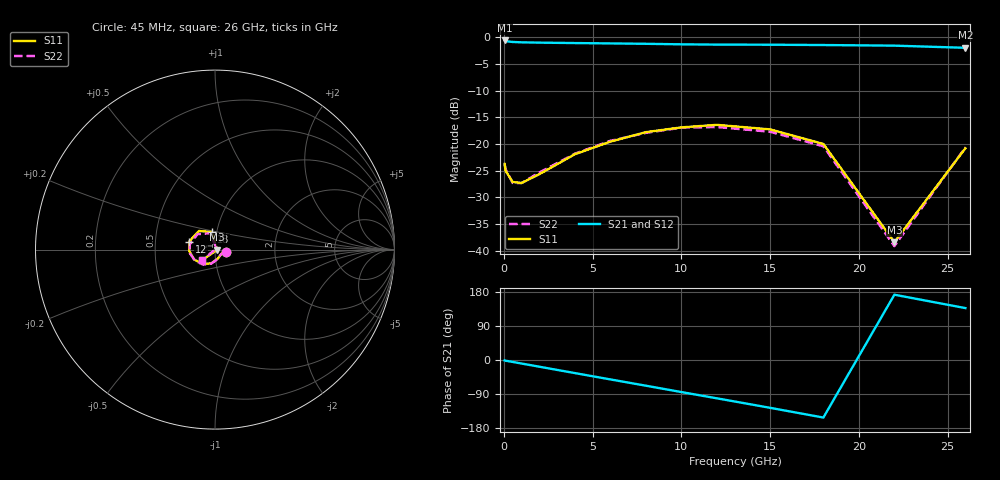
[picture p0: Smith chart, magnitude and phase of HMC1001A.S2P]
! HMMC-1001
! Typical s-parameters at minimum attenuation setting, Ta=25øC
# ghz s ma r 50
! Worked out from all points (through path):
!   14 points, 45 MHz to 26 GHz, reference 50 ohm
!   highest |S21| = -0.59 dB at 45 MHz (marker M1); lowest = -2.0 dB at 26 GHz (marker M2)
!   lowest |S11| = -38.4 dB at 22 GHz (marker M3), VSWR 1.02, Z = 51.2 - j0.109 ohm
!   |S11| at or under -10 dB: start of sweep to end of sweep
!   |S22| runs from -39.2 to -16.8 dB; largest |S21 - S12| = 0.016
!   S11 on the Smith chart (normalised r, x): 45 MHz: 1.14, -0.03; 12 GHz: 0.75, +0.07; 18 GHz: 0.94, +0.19; 26 GHz: 0.86, -0.10
0.045  0.065 -11.0  0.934 -1.0  0.932 -1.2  0.065 -12.5
0.1  0.056 -18.0  0.921 -1.9  0.92 -1.8  0.058 -18.9
0.5  0.044 -30.4  0.904 -5.1  0.903 -5.0  0.043 -30.0
1  0.043 -45.3  0.897 -9.3  0.896 -9.2  0.043 -46.5
2  0.052 -71.0  0.891 -17.7  0.891 -17.6  0.054 -71.3
4  0.08 -105.8  0.883 -34.5  0.883 -34.4  0.081 -104.9
6  0.105 -131.1  0.876 -51.2  0.876 -51.2  0.107 -127.9
8  0.129 -154.7  0.869 -67.8  0.866 -68.0  0.127 -151.1
10  0.143 -176.5  0.859 -84.6  0.86 -84.6  0.142 -171.6
12  0.151 162.7  0.854 -101.1  0.856 -101.0  0.144 168.7
15  0.137 130.8  0.852 -126.2  0.852 -126.4  0.13 138.7
18  0.1 101.1  0.846 -151.9  0.847 -152.0  0.095 106.8
22  0.012 -5.1  0.835 172.3  0.831 172.8  0.011 34.2
26  0.091 -140.5  0.797 137.0  0.794 135.9  0.093 -142.0
